FUNCTION "CONTROL_FLASH.OFF" : VOID
TITLE =
{ S7_language := '9(1) Inglese (Stati Uniti)  11.01.2022  09:45:15' }
VERSION : 0.1

BEGIN
NETWORK
TITLE =********** BURNER 01 ************



NETWORK
TITLE =PID PARAMETERS
//CONTROL LOOP BURNER
//----------------------------------------------------
//ACTUATOR: BURNER 1
//FEEDBACK: ..........
//----------------------------------------------------
//
//PID SETUP
      L     1.000000e-001; //(0,1 SEC)
      T     "DBI_PID_BRN1".CYCLE;
      L     3.000000e+001; //(10 SEC.)
      T     "DBI_PID_BRN1".MTR_TM;
      L     1.000000e+000; //(1 SEC.)
      T     "DBI_PID_BRN1".PULSE_TM;
      L     5.000000e-001; //(1 SEC.)
      T     "DBI_PID_BRN1".BREAK_TM;

//DATA FROM SCADA
      L     "DB_GRP_80_R30".TIC71_IN_GR1_PID.PV.DeadBand_SP;
      T     "DBI_PID_BRN1".DEADB_W;

      L     "DBI_PID_BRN1".DEADB_W;
      L     0.000000e+000;
      >R    ;
      SPB   M005;
      L     0.000000e+000;
      T     "DBI_PID_BRN1".DEADB_W;
      T     "DB_GRP_80_R30".TIC71_IN_GR1_PID.PV.DeadBand_SP;
M005: NOP   0;

      L     "DB_GRP_80_R30".TIC71_IN_GR1_PID.PV.PropGain_SP;
      T     "DBI_PID_BRN1".GAIN;

      L     "DBI_PID_BRN1".GAIN;
      L     0.000000e+000;
      >R    ;
      SPB   M003;
      L     3.000000e+000;
      T     "DBI_PID_BRN1".GAIN;
      T     "DB_GRP_80_R30".TIC71_IN_GR1_PID.PV.PropGain_SP;
M003: NOP   0;

      L     "DB_GRP_80_R30".TIC71_IN_GR1_PID.PV.IntegralTime_SP;
      T     "DBI_PID_BRN1".TI;

      L     "DBI_PID_BRN1".TI;
      L     0.000000e+000;
      >R    ;
      SPB   M004;
      L     6.000000e+001;
      T     "DBI_PID_BRN1".TI;
      T     "DB_GRP_80_R30".TIC71_IN_GR1_PID.PV.IntegralTime_SP;
M004: NOP   0;

      L     0.000000e+000;
      T     "DBI_PID_BRN1".DISV;

NETWORK
TITLE =MOVE TEMPERATURE SETPOINT
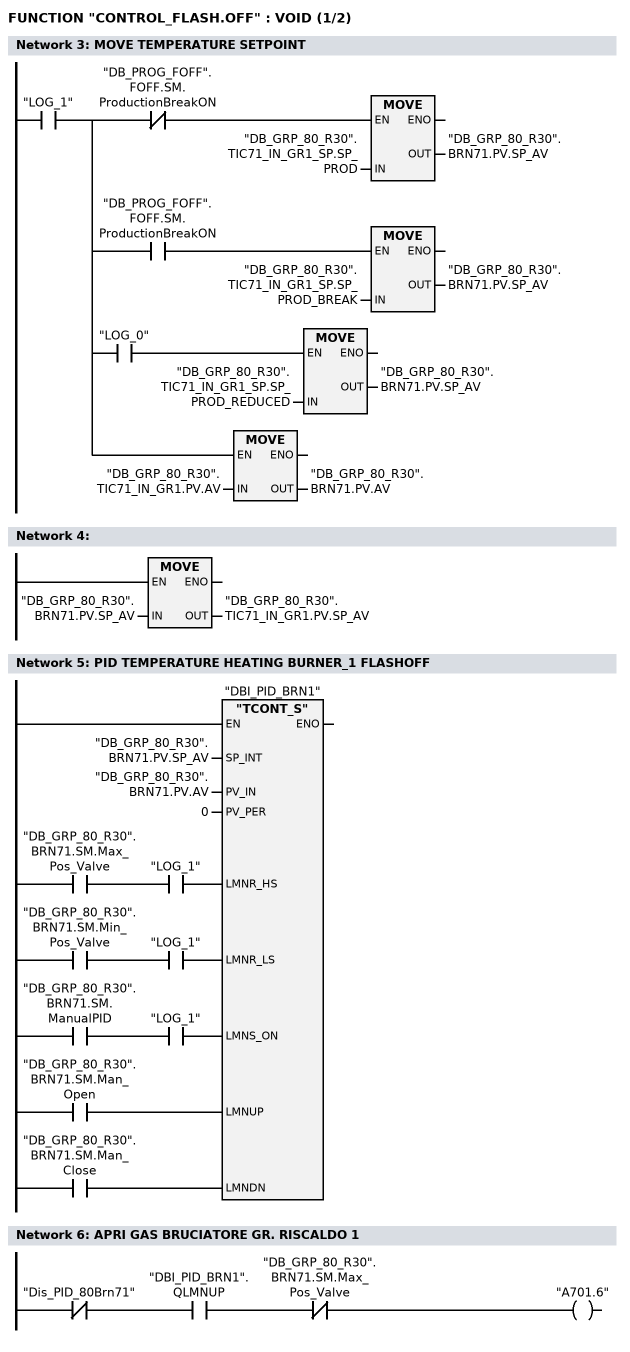
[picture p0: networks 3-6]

      U     "LOG_1";
      =     L      0.0;
      U     L      0.0;
      UN    "DB_PROG_FOFF".FOFF.SM.ProductionBreakON;
      SPBNB _001;
      L     "DB_GRP_80_R30".TIC71_IN_GR1_SP.SP_PROD;
      T     "DB_GRP_80_R30".BRN71.PV.SP_AV;
_001: NOP   0;
      U     L      0.0;
      U     "DB_PROG_FOFF".FOFF.SM.ProductionBreakON;
      SPBNB _002;
      L     "DB_GRP_80_R30".TIC71_IN_GR1_SP.SP_PROD_BREAK;
      T     "DB_GRP_80_R30".BRN71.PV.SP_AV;
_002: NOP   0;
      U     L      0.0;
      U     "LOG_0";
      SPBNB _003;
      L     "DB_GRP_80_R30".TIC71_IN_GR1_SP.SP_PROD_REDUCED;
      T     "DB_GRP_80_R30".BRN71.PV.SP_AV;
_003: NOP   0;
      U     L      0.0;
      SPBNB _004;
      L     "DB_GRP_80_R30".TIC71_IN_GR1.PV.AV;
      T     "DB_GRP_80_R30".BRN71.PV.AV;
_004: NOP   0;
NETWORK
TITLE =

      L     "DB_GRP_80_R30".BRN71.PV.SP_AV;
      T     "DB_GRP_80_R30".TIC71_IN_GR1.PV.SP_AV;
      NOP   0;
NETWORK
TITLE = PID TEMPERATURE HEATING BURNER_1 FLASHOFF

      U     "DB_GRP_80_R30".BRN71.SM.Max_Pos_Valve;
      U     "LOG_1";
      =     L      0.0;
      BLD   103;
      U     "DB_GRP_80_R30".BRN71.SM.Min_Pos_Valve;
      U     "LOG_1";
      =     L      0.1;
      BLD   103;
      U     "DB_GRP_80_R30".BRN71.SM.ManualPID;
      U     "LOG_1";
      =     L      0.2;
      BLD   103;
      U     "DB_GRP_80_R30".BRN71.SM.Man_Open;
      =     L      0.3;
      BLD   103;
      U     "DB_GRP_80_R30".BRN71.SM.Man_Close;
      =     L      0.4;
      BLD   103;
      CALL "TCONT_S" , "DBI_PID_BRN1" (
           SP_INT                   := "DB_GRP_80_R30".BRN71.PV.SP_AV,
           PV_IN                    := "DB_GRP_80_R30".BRN71.PV.AV,
           PV_PER                   := 0,
           LMNR_HS                  := L      0.0,
           LMNR_LS                  := L      0.1,
           LMNS_ON                  := L      0.2,
           LMNUP                    := L      0.3,
           LMNDN                    := L      0.4);

      NOP   0;
NETWORK
TITLE = APRI GAS BRUCIATORE GR. RISCALDO 1

      UN    "Dis_PID_80Brn71";
      U     "DBI_PID_BRN1".QLMNUP;
      UN    "DB_GRP_80_R30".BRN71.SM.Max_Pos_Valve;
      =     "A701.6";
NETWORK
TITLE = CHIUDI GAS BRUCIATORE GR. RISCALDO 1
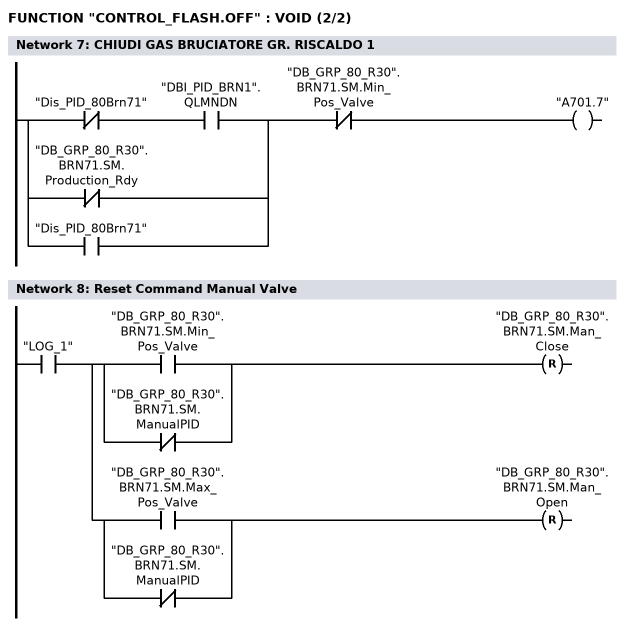
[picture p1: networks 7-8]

      U(    ;
      UN    "Dis_PID_80Brn71";
      U     "DBI_PID_BRN1".QLMNDN;
      ON    "DB_GRP_80_R30".BRN71.SM.Production_Rdy;
      O     "Dis_PID_80Brn71";
      )     ;
      UN    "DB_GRP_80_R30".BRN71.SM.Min_Pos_Valve;
      =     "A701.7";
NETWORK
TITLE =Reset Command Manual Valve

      U     "LOG_1";
      =     L      0.0;
      U     L      0.0;
      U(    ;
      O     "DB_GRP_80_R30".BRN71.SM.Min_Pos_Valve;
      ON    "DB_GRP_80_R30".BRN71.SM.ManualPID;
      )     ;
      R     "DB_GRP_80_R30".BRN71.SM.Man_Close;
      U     L      0.0;
      U(    ;
      O     "DB_GRP_80_R30".BRN71.SM.Max_Pos_Valve;
      ON    "DB_GRP_80_R30".BRN71.SM.ManualPID;
      )     ;
      R     "DB_GRP_80_R30".BRN71.SM.Man_Open;
NETWORK
TITLE =



NETWORK
TITLE =PID PARAMETERS
//CONTROL LOOP BURNER
//----------------------------------------------------
//ACTUATOR: BURNER 2
//FEEDBACK: ..........
//----------------------------------------------------
//
//PID SETUP
      L     1.000000e-001; //(0,1 SEC)
      T     "DBI_PID_BRN2".CYCLE;
      L     3.000000e+001; //(30 SEC.)
      T     "DBI_PID_BRN2".MTR_TM;
      L     1.000000e+000; //(1 SEC.)
      T     "DBI_PID_BRN2".PULSE_TM;
      L     5.000000e-001; //(1 SEC.)
      T     "DBI_PID_BRN2".BREAK_TM;

//DATA FROM SCADA
      L     "DB_GRP_80_R30".TIC71_IN_GR2_PID.PV.DeadBand_SP;
      T     "DBI_PID_BRN2".DEADB_W;

      L     "DBI_PID_BRN2".DEADB_W;
      L     0.000000e+000;
      >R    ;
      SPB   M008;
      L     0.000000e+000;
      T     "DBI_PID_BRN2".DEADB_W;
      T     "DB_GRP_80_R30".TIC71_IN_GR2_PID.PV.DeadBand_SP;
M008: NOP   0;

      L     "DB_GRP_80_R30".TIC71_IN_GR2_PID.PV.PropGain_SP;
      T     "DBI_PID_BRN2".GAIN;

      L     "DBI_PID_BRN2".GAIN;
      L     0.000000e+000;
      >R    ;
      SPB   M009;
      L     3.000000e+000;
      T     "DBI_PID_BRN2".GAIN;
      T     "DB_GRP_80_R30".TIC71_IN_GR2_PID.PV.PropGain_SP;
M009: NOP   0;

      L     "DB_GRP_80_R30".TIC71_IN_GR2_PID.PV.IntegralTime_SP;
      T     "DBI_PID_BRN2".TI;

      L     "DBI_PID_BRN2".TI;
      L     0.000000e+000;
      >R    ;
      SPB   M00a;
      L     6.000000e+001;
      T     "DBI_PID_BRN2".TI;
      T     "DB_GRP_80_R30".TIC71_IN_GR2_PID.PV.IntegralTime_SP;
M00a: NOP   0;

      L     0;
      T     "DBI_PID_BRN2".DISV;


NETWORK
TITLE =MOVE TEMPERATURE SETPOINT
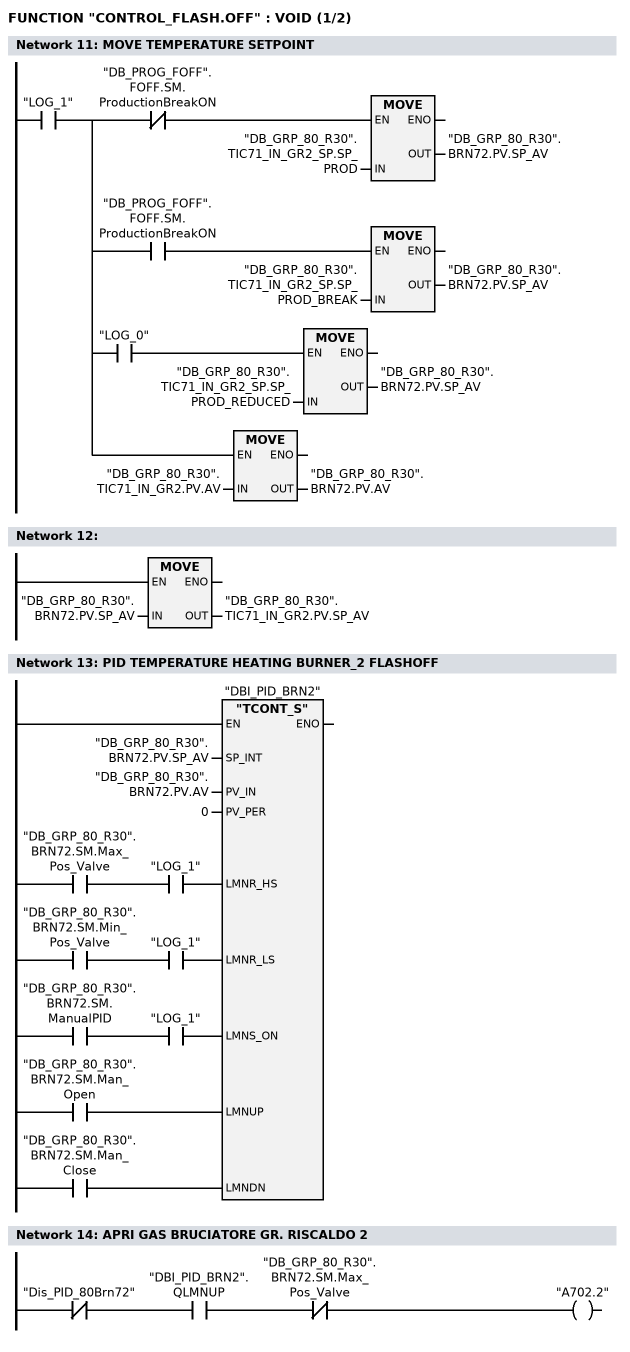
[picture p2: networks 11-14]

      U     "LOG_1";
      =     L      0.0;
      U     L      0.0;
      UN    "DB_PROG_FOFF".FOFF.SM.ProductionBreakON;
      SPBNB _005;
      L     "DB_GRP_80_R30".TIC71_IN_GR2_SP.SP_PROD;
      T     "DB_GRP_80_R30".BRN72.PV.SP_AV;
_005: NOP   0;
      U     L      0.0;
      U     "DB_PROG_FOFF".FOFF.SM.ProductionBreakON;
      SPBNB _006;
      L     "DB_GRP_80_R30".TIC71_IN_GR2_SP.SP_PROD_BREAK;
      T     "DB_GRP_80_R30".BRN72.PV.SP_AV;
_006: NOP   0;
      U     L      0.0;
      U     "LOG_0";
      SPBNB _007;
      L     "DB_GRP_80_R30".TIC71_IN_GR2_SP.SP_PROD_REDUCED;
      T     "DB_GRP_80_R30".BRN72.PV.SP_AV;
_007: NOP   0;
      U     L      0.0;
      SPBNB _008;
      L     "DB_GRP_80_R30".TIC71_IN_GR2.PV.AV;
      T     "DB_GRP_80_R30".BRN72.PV.AV;
_008: NOP   0;
NETWORK
TITLE =

      L     "DB_GRP_80_R30".BRN72.PV.SP_AV;
      T     "DB_GRP_80_R30".TIC71_IN_GR2.PV.SP_AV;
      NOP   0;
NETWORK
TITLE = PID TEMPERATURE HEATING BURNER_2 FLASHOFF

      U     "DB_GRP_80_R30".BRN72.SM.Max_Pos_Valve;
      U     "LOG_1";
      =     L      0.0;
      BLD   103;
      U     "DB_GRP_80_R30".BRN72.SM.Min_Pos_Valve;
      U     "LOG_1";
      =     L      0.1;
      BLD   103;
      U     "DB_GRP_80_R30".BRN72.SM.ManualPID;
      U     "LOG_1";
      =     L      0.2;
      BLD   103;
      U     "DB_GRP_80_R30".BRN72.SM.Man_Open;
      =     L      0.3;
      BLD   103;
      U     "DB_GRP_80_R30".BRN72.SM.Man_Close;
      =     L      0.4;
      BLD   103;
      CALL "TCONT_S" , "DBI_PID_BRN2" (
           SP_INT                   := "DB_GRP_80_R30".BRN72.PV.SP_AV,
           PV_IN                    := "DB_GRP_80_R30".BRN72.PV.AV,
           PV_PER                   := 0,
           LMNR_HS                  := L      0.0,
           LMNR_LS                  := L      0.1,
           LMNS_ON                  := L      0.2,
           LMNUP                    := L      0.3,
           LMNDN                    := L      0.4);

      NOP   0;
NETWORK
TITLE = APRI GAS BRUCIATORE GR. RISCALDO 2

      UN    "Dis_PID_80Brn72";
      U     "DBI_PID_BRN2".QLMNUP;
      UN    "DB_GRP_80_R30".BRN72.SM.Max_Pos_Valve;
      =     "A702.2";
NETWORK
TITLE = CHIUDI GAS BRUCIATORE GR. RISCALDO 2
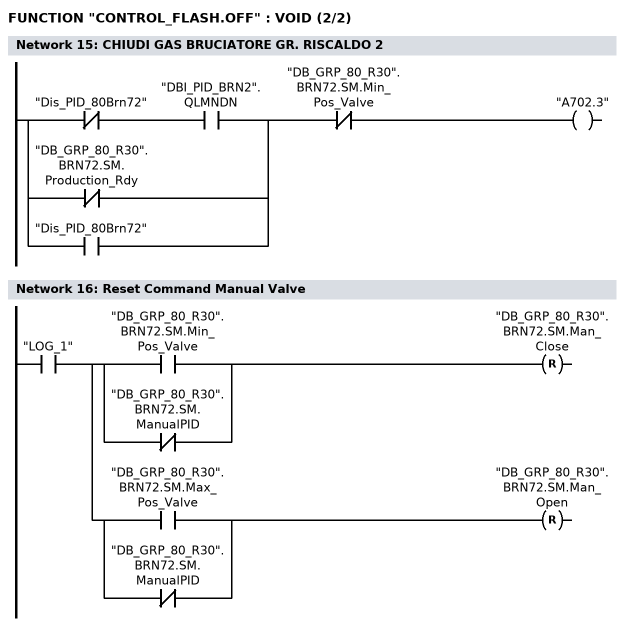
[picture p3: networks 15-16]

      U(    ;
      UN    "Dis_PID_80Brn72";
      U     "DBI_PID_BRN2".QLMNDN;
      ON    "DB_GRP_80_R30".BRN72.SM.Production_Rdy;
      O     "Dis_PID_80Brn72";
      )     ;
      UN    "DB_GRP_80_R30".BRN72.SM.Min_Pos_Valve;
      =     "A702.3";
NETWORK
TITLE =Reset Command Manual Valve

      U     "LOG_1";
      =     L      0.0;
      U     L      0.0;
      U(    ;
      O     "DB_GRP_80_R30".BRN72.SM.Min_Pos_Valve;
      ON    "DB_GRP_80_R30".BRN72.SM.ManualPID;
      )     ;
      R     "DB_GRP_80_R30".BRN72.SM.Man_Close;
      U     L      0.0;
      U(    ;
      O     "DB_GRP_80_R30".BRN72.SM.Max_Pos_Valve;
      ON    "DB_GRP_80_R30".BRN72.SM.ManualPID;
      )     ;
      R     "DB_GRP_80_R30".BRN72.SM.Man_Open;
NETWORK
TITLE =



NETWORK
TITLE =
//CONTROL LOOP COOLER FLASH-OFF
//----------------------------------------------------
//ACTUATOR: COLD VALVE
//FEEDBACK: ..........
//----------------------------------------------------
//
NETWORK
TITLE =



NETWORK
TITLE =manual operation on

      U     "LOG_1";
      =     L      0.0;
      U     L      0.0;
      U     "DB_GRP_80_R30".VM71_VALVE.SM.ManualMode;
      =     "DBI_PID_FSHOFF_COOL".MAN_ON;
      U     L      0.0;
      UN    "DB_GRP_80_R30".VM71_VALVE.SM.ManualMode;
      U     "DB_GRP_80_R30".VM71_VALVE.SM.ManualMode;
      SPBNB _009;
      L     0.000000e+000;
      T     "DB_GRP_80_R30".VM71_VALVE.PV.Man_Position;
_009: NOP   0;
      U     L      0.0;
      SPBNB _00a;
      L     "DB_GRP_80_R30".VM71_VALVE.PV.Man_Position;
      T     "DBI_PID_FSHOFF_COOL".MAN;
_00a: NOP   0;
      U(    ;
      U     L      0.0;
      SPBNB _00b;
      L     "DBI_PID_FSHOFF_COOL".LMN;
      T     "DB_GRP_80_R30".VM71_VALVE.PV.Position;
      SET   ;
      SAVE  ;
      CLR   ;
_00b: U     BIE;
      )     ;
      SPBNB _00c;
      L     "DBI_PID_FSHOFF_COOL".LMN;
      T     "DB_GRP_80_R30".TIC75_IN_COOL_PID.PV.ManipulatedVariable_AV;
_00c: NOP   0;
NETWORK
TITLE =CONTROLLER ON / CONTROLLER OFF

      O     "DB_GRP_80_R30".FAN73.SM.MotorOn;
      O     "DB_GRP_80_R30".VM71_VALVE.SM.ManualMode;
      =     L      0.0;
      U     L      0.0;
      BLD   102;
      =     "DB_GRP_80_R30".TIC75_IN_COOL_PID.SM.CTRL_On;
      U     L      0.0;
      BLD   102;
      =     "DB_GRP_80_R30".VM71_VALVE.SM.Enabled;
      U     L      0.0;
      NOT   ;
      =     "DB_GRP_80_R30".TIC75_IN_COOL_PID.SM.CTRL_Off;
NETWORK
TITLE =


      L     1.000000e+002;
      UN    "DB_GRP_80_R30".TIC75_IN_COOL_PID.SM.CTRL_Off;
      SPB   M012;
      L     0.000000e+000;
M012: T     "DBI_PID_FSHOFF_COOL".LMN_HLM;


NETWORK
TITLE =Valvola Freddo Cooler

//PID SETUP
      L     1.000000e-001;
      T     "DBI_PID_FSHOFF_COOL".CYCLE;

      L     0.000000e+000;
      T     "DBI_PID_FSHOFF_COOL".LMN_LLM;

      L     1.000000e+002;
      T     "DBI_PID_FSHOFF_COOL".LMN_HLM;

//DATA FROM VISUALISATION
      L     "DB_GRP_80_R30".TIC75_IN_COOL_PID.PV.DeadBand_SP;
      T     "DBI_PID_FSHOFF_COOL".DEADB_W;

      L     "DB_GRP_80_R30".TIC75_IN_COOL_PID.PV.PropGain_SP;
      L     0.000000e+000;
      >R    ;
      SPB   _03;
      L     3.000000e+000;
      T     "DB_GRP_80_R30".TIC75_IN_COOL_PID.PV.PropGain_SP;

_03:  L     "DB_GRP_80_R30".TIC75_IN_COOL_PID.PV.PropGain_SP;
      L     -1.000000e+000;
      *R    ;
      T     "DBI_PID_FSHOFF_COOL".GAIN;

      L     "DB_GRP_80_R30".TIC75_IN_COOL_PID.PV.IntegralTime_SP;
      T     "DBI_PID_FSHOFF_COOL".TI;

      L     "DB_GRP_80_R30".TIC75_IN_COOL_PID.PV.DerivativeTime_SP;
      T     "DBI_PID_FSHOFF_COOL".TD;

// CONTROL LOOP SIGNALS
      L     "DB_GRP_80_R30".TIC75_IN_COOL.PV.AV;
      T     "DB_GRP_80_R30".VM71_VALVE.PV.AV;
      T     "DBI_PID_FSHOFF_COOL".PV_IN;

      L     "DB_GRP_80_R30".TIC75_IN_COOL_SP.SP_PROD;
      T     "DB_GRP_80_R30".TIC75_IN_COOL.PV.SP_AV;
      T     "DB_GRP_80_R30".VM71_VALVE.PV.SP_AV;
      T     "DBI_PID_FSHOFF_COOL".SP_INT;



NETWORK
TITLE =PID COLD VALVE FALSH-OFF
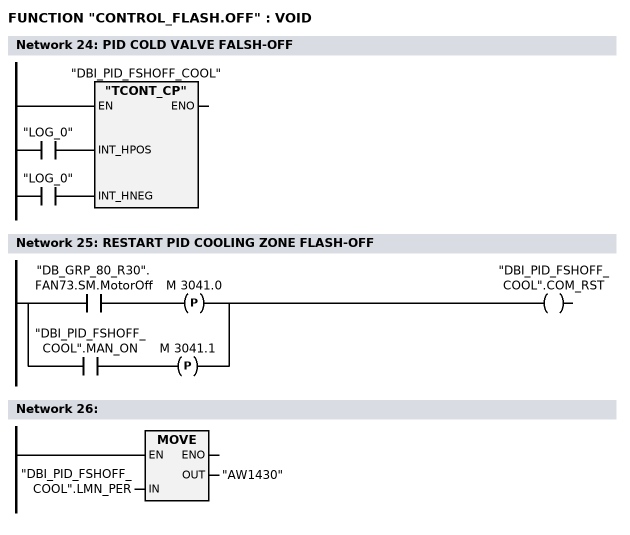
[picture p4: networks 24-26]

      U     "LOG_0";
      =     L      0.0;
      BLD   103;
      U     "LOG_0";
      =     L      0.1;
      BLD   103;
      CALL "TCONT_CP" , "DBI_PID_FSHOFF_COOL" (
           INT_HPOS                 := L      0.0,
           INT_HNEG                 := L      0.1);

      NOP   0;
NETWORK
TITLE =RESTART PID COOLING ZONE FLASH-OFF

      U     "DB_GRP_80_R30".FAN73.SM.MotorOff;
      FP    M   3041.0;
      O(    ;
      U     "DBI_PID_FSHOFF_COOL".MAN_ON;
      FP    M   3041.1;
      )     ;
      =     "DBI_PID_FSHOFF_COOL".COM_RST;
NETWORK
TITLE =

      L     "DBI_PID_FSHOFF_COOL".LMN_PER;
      T     "AW1430";
      NOP   0;
NETWORK
TITLE =



END_FUNCTION

